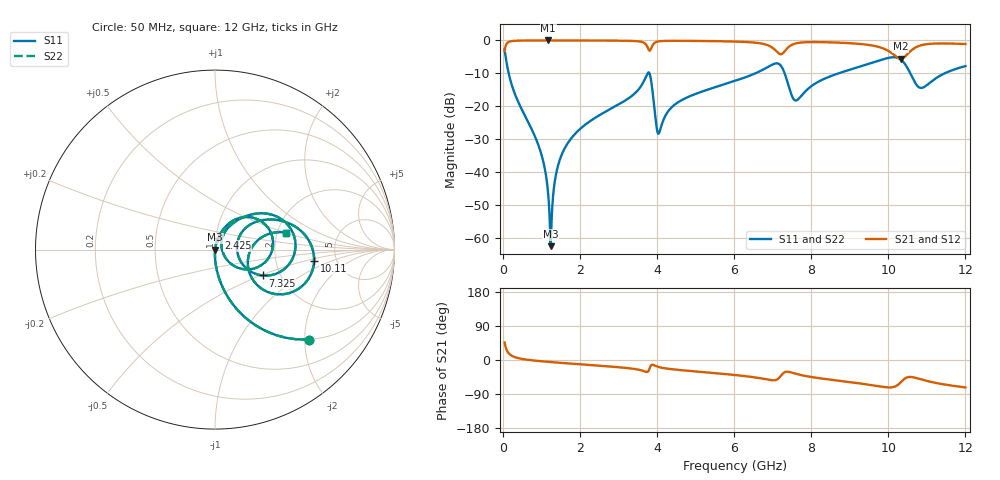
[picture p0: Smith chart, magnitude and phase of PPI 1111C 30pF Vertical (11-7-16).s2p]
# GHz S MA R 50
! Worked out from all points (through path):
!   1601 points, 50 MHz to 12 GHz, reference 50 ohm
!   highest |S21| = -0.01 dB at 1.178 GHz (marker M1); lowest = -5.5 dB at 10.33 GHz (marker M2)
!   group delay of S21, straight-line fit = 17.2 ps
!   lowest |S11| = -62.4 dB at 1.245 GHz (marker M3), VSWR 1.00, Z = 50.1 - j0.00251 ohm
!   |S11| at or under -10 dB: 156 MHz to 3.757 GHz (3.601 GHz wide, 184 % of centre); 3.808 GHz to 6.549 GHz (2.741 GHz wide, 52.9 % of centre); 7.313 GHz to 8.707 GHz (1.394 GHz wide, 17.4 % of centre)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
!   |S22| runs from -62.4 to -2.8 dB; largest |S21 - S12| = 0
!   S11 on the Smith chart (normalised r, x): 50 MHz: 0.99, -2.10; 2.425 GHz: 1.03, +0.14; 7.325 GHz: 1.62, -0.52; 10.11 GHz: 3.37, -0.63; 12 GHz: 2.24, +0.51
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0.05  0.7256 -43.7  0.688 46.3  0.688 46.3  0.7256 -43.7
0.2367188  0.2103 -78.8  0.9772 11.1  0.9772 11.1  0.2103 -78.8
0.9835938  0.02047 -91.2  0.9991 -3.1  0.9991 -3.1  0.02047 -91.2
1.177781  0.004832 -86.1  0.9992 -4.8  0.9992 -4.8  0.004832 -86.1
1.245  0.0007558 -1.9  0.9992 -5.4  0.9992 -5.4  0.0007558 -1.9
1.491469  0.01608 79.7  0.999 -7.4  0.999 -7.4  0.01608 79.7
2.044156  0.04739 77.2  0.9977 -11.6  0.9977 -11.6  0.04739 77.2
2.425063  0.06853 74.6  0.9962 -14.4  0.9962 -14.4  0.06853 74.6
3.463219  0.1648 62.0  0.9756 -24.4  0.9756 -24.4  0.1648 62.0
3.776906  0.3263 15.5  0.7422 -29.6  0.7422 -29.6  0.3263 15.5
4.038312  0.03832 10.5  0.966 -18.4  0.966 -18.4  0.03832 10.5
4.546188  0.115 60.7  0.9866 -26.0  0.9866 -26.0  0.115 60.7
6.025  0.2433 48.4  0.9612 -39.6  0.9612 -39.6  0.2433 48.4
6.876437  0.395 27.2  0.8458 -51.8  0.8458 -51.8  0.395 27.2
7.324562  0.3025 -28.5  0.6974 -31.7  0.6974 -31.7  0.3025 -28.5
7.585969  0.1229 -0.7  0.8965 -35.8  0.8965 -35.8  0.1229 -0.7
8.019156  0.2052 35.1  0.9441 -45.2  0.9441 -45.2  0.2052 35.1
10.01331  0.5449 -0.2  0.688 -72.4  0.688 -72.4  0.5449 -0.2
10.11041  0.5556 -6.6  0.6294 -71.8  0.6294 -71.8  0.5556 -6.6
10.327  0.5119 -25.5  0.5303 -58.5  0.5303 -58.5  0.5119 -25.5
10.84234  0.1903 -13.2  0.8421 -50.9  0.8421 -50.9  0.1903 -13.2
12  0.4077 13.4  0.8829 -72.4  0.8829 -72.4  0.4077 13.4
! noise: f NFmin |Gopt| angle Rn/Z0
0.05  0.0003319  0.852  0.9991  0.0004783
1.372  0.003255  0.6331  5.89  0.001664
2.701  0.00643  0.6359  11.14  0.003297
4.031  0.0368  0.8913  17.28  0.07203
5.36  0.0158  0.7014  22.13  0.009997
6.682  0.04827  0.8683  27.97  0.07424
8.012  0.05108  0.8546  33.31  0.06888
9.341  0.05606  0.8494  38.23  0.07081
10.67  0.167  0.9407  43.56  0.5431
12  0.05785  0.824  47.88  0.05776
